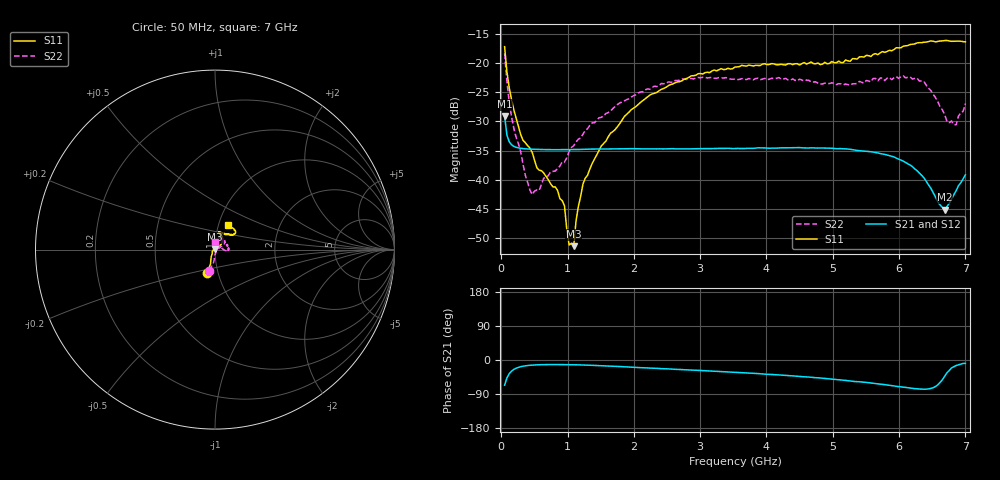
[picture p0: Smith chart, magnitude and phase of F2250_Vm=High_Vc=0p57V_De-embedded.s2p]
! Integrated Device Technology
! Corporate Headquarters
! 6024 Silver Creek Valley Road
! San Jose, CA 95138  USA
! Phone:  1-408-284-8200
! Toll Free:  1-800-223-1366
! Webpage:  http://www.idt.com/
! Timing and RF Division
! 515 Groton Road, Suite 102
! Westford, MA 01886-6024
! Device:  F2250
! Description: Voltage Variable RF Attenuator
! Frequency:  50.0 -  6000.00 MHz
! Package:  3x3 mm Thin QFN Plastic Package: 16 pin
! Ports:  2 RF, 3 DC
!  Pin  1  = GND
!  Pin  2  = NC
!  Pin  3  = RF1  = Port 1
!  Pin  4  = NC
!  Pin  5  = GND
!  Pin  6  = GND
!  Pin  7  = GND
!  Pin  8  = GND
!  Pin  9  = NC
!  Pin 10  = RF2  = Port 2
!  Pin 11  = NC
!  Pin 12  = GND
!  Pin 13  = GND
!  Pin 14  = VCNTRL
!  Pin 15  = VDD
!  Pin 16  = VMODE
! Vcntrl:  0.570 Volts
! Vmode:  +3.300 Volts
! Vdd:  +3.30  Volts
! Current:  1.273 mA
! Data:  The device was measured on a the F2250 evaluation board which has
!  individual transmission lines to the RF pins.  Data was collected
!  using a calibrated network analyzer.  The evaluation board was
!  de-embedded using a TRL calibration technique.
!  The reference plane is the edge of the package pin.
! Misc:  SN 10
!  Action Tracker AT0258
! Date Measured:  2014-11-26
! Date:  2015-10-15  MJV
! Note:
!  Integrated Device Technology supplies this data as a sample of measured
!  data at the package pin for this product.  Your particular data for this
!  product may vary.
!  Data was taken at 25 degrees C.
!  Integrated Device Technology reserves the right to change this data at anytime.
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# GHz S dB R 50
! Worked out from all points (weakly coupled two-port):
!   201 points, 50 MHz to 7 GHz, reference 50 ohm
!   highest |S21| = -29.10 dB at 50 MHz (marker M1); lowest = -45.1 dB at 6.687 GHz (marker M2)
!   lowest |S11| = -51.4 dB at 1.093 GHz (marker M3), VSWR 1.01, Z = 50 + j0.268 ohm
!   |S11| at or under -10 dB: start of sweep to end of sweep
!   |S22| runs from -42.5 to -18.4 dB; largest |S21 - S12| = 5.2e-05
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0.05  -17.17 -108.4  -29.10 -66.5  -29.10 -66.5  -18.35 -105.2
0.08475  -21.47 -107.3  -32.34 -47.5  -32.34 -47.5  -23.13 -95.8
0.15425  -26.23 -116.4  -34.01 -29.3  -34.01 -29.3  -29.20 -92.7
0.29325  -32.29 -127.1  -34.62 -17.7  -34.62 -17.7  -35.23 -72.5
0.36275  -33.67 -139.2  -34.71 -15.4  -34.71 -15.4  -39.25 -55.6
0.467  -35.34 -145.7  -34.78 -13.5  -34.78 -13.5  -42.55 -32.2
0.5365  -37.95 -154.1  -34.81 -12.8  -34.80 -12.8  -41.75 -17.1
0.91875  -43.59 155.8  -34.86 -12.2  -34.86 -12.2  -36.94 13.5
0.9535  -44.51 171.4  -34.86 -12.2  -34.86 -12.2  -36.96 21.0
1.023  -51.22 139.6  -34.85 -12.4  -34.85 -12.3  -35.14 21.4
1.0925  -51.42 85.1  -34.84 -12.5  -34.84 -12.5  -34.18 23.4
1.12725  -47.10 59.7  -34.83 -12.7  -34.83 -12.7  -33.55 21.2
1.2315  -40.78 39.8  -34.80 -13.1  -34.79 -13.2  -32.20 18.8
1.6485  -32.02 40.7  -34.73 -16.1  -34.73 -16.1  -28.24 27.2
2.37825  -24.75 46.5  -34.71 -22.4  -34.71 -22.4  -23.85 35.1
3.525  -20.66 71.6  -34.67 -32.5  -34.67 -32.5  -22.74 61.7
4.7065  -20.07 71.9  -34.54 -46.1  -34.55 -46.1  -23.23 63.4
5.85325  -17.80 40.5  -35.90 -66.7  -35.90 -66.9  -22.43 12.7
6.3745  -16.41 40.9  -39.68 -77.1  -39.70 -77.2  -23.13 -3.8
6.68725  -16.12 47.8  -45.13 -42.7  -45.11 -42.4  -28.83 17.9
6.861  -16.22 54.5  -41.89 -14.5  -41.88 -14.6  -30.58 59.6
7  -16.34 62.4  -39.18 -8.8  -39.15 -8.9  -26.92 93.2
